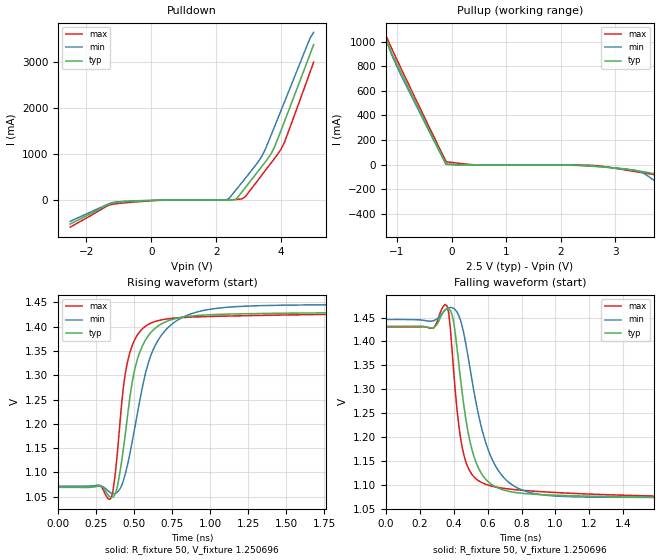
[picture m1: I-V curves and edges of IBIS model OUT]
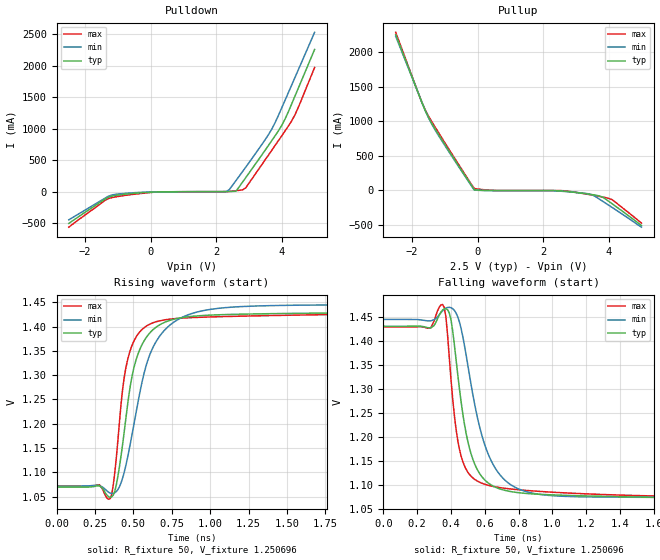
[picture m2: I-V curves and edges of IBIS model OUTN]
|   IBIS File of SG2520VGN D
|   LVDS, Vcc=2.5V, Io=3.5mA, fo<=212.5MHz
[IBIS Ver]   3.2
[File Name]   sg2520vgn_35m_25v.ibs
[File Rev]   1.0
[Date]   Sep. 11, 2020
[Source]
Fairchild Ensigna Lab's Method
[Notes]
Created by Minoru Kozaki
[Disclaimer]
Seiko Epson Corporation makes no warranty with respect to the
information contained herein.
[Copyright]
Copyright(C) 2020, Seiko Epson Corporation. All rights reserved.
|   Component
[Component]   SG2520VGN
[Manufacturer]  Seiko Epson Corporation
[Package]
R_pkg   17.7m   NA   NA
L_pkg   235p   NA   NA
C_pkg   208f   NA   NA
[Pin]   signal_name   model_name   R_pin   L_pin   C_pin
1   OE/ST   NC
2   NC   NC
3   GND   GND
4   OUT   OUT   17.7m   235p   208f
5   OUTN   OUTN   10.4m   129p   221f
6   VCC   POWER
[Diff Pin] inv_pin  vdiff  tdelay_typ
4   5   0   0
| Models and submodels in the file (2): OUT (Output), OUTN (Output)
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|   Model OUT
[Model]   OUT
Model_type   Output
Polarity   Non-Inverting
Vref = 1.25
Vmeas = 1.25
Rref = 50
Cref = 0
C_comp   4.5p   4.5p   4.5p
[Temperature Range]   25   105   -40
[Voltage Range]   2.5   2.25   2.75
[Pullup Reference]   2.5   2.25   2.75
[Pulldown Reference]   0   0   0
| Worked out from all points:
|   slope of the pulldown table from 0 to 0.375 V, typ, clamps not added: 66 ohm
|   slope of the pullup table from 0 to 0.375 V, typ, clamps not added: 55.5 ohm
|   falling waveform, R_fixture 50, V_fixture 1.250696: 20-80 % time 109ps typ, 153ps min, 81.3ps max; typ from 1.43 V to 1.07 V
|   rising waveform, R_fixture 50, V_fixture 1.250696: 20-80 % time 126ps typ, 178ps min, 93.2ps max; typ from 1.07 V to 1.43 V
[Pullup]
-2.5V     3.361A     3.265A     3.472A
-1.3V     1.161A     1.17A      1.172A
-1.2V     1.019A     1.015A     1.048A
-1V       817.6mA    797.6mA    853.4mA
-100mV    7.392mA    1.916mA    24.92mA
500mV     -3.42mA    -3.608mA   -2.547mA
2.6V      -11.61mA   -13.33mA   -5.781mA
3.4V      -49.69mA   -49.62mA   -58.4mA
3.5V      -56.25mA   -65.55mA   -65.49mA
3.8V      -93.02mA   -157.5mA   -88.11mA
4.1V      -200.5mA   -252.7mA   -132mA
5V        -521.7mA   -541.9mA   -494.1mA
[Pulldown]
-2.5V     -513.3mA   -455.2mA   -580.8mA
-1.2V     -62.9mA    -49.06mA   -86.29mA
200mV     414.9uA    905.7uA    -721.7uA
2.4V      5.862mA    46.91mA    8.441mA
2.6V      12.01mA    219mA      19.18mA
2.9V      278.6mA    480.8mA    81.84mA
3.4V      729mA      948.8mA    543mA
3.7V      1.021A     1.429A     819.6mA
4V        1.522A     1.952A     1.112A
4.1V      1.705A     2.126A     1.256A
4.8V      2.997A     3.356A     2.599A
5V        3.369A     3.636A     2.99A
[Falling Waveform]
R_fixture = 50
V_fixture = 1.250696
V_fixture_min = 1.258555
V_fixture_max = 1.251296
0s        1.432V     1.446V     1.43V
280ps     1.428V     1.443V     1.427V
360ps     1.468V     1.469V     1.474V
380ps     1.465V     1.471V     1.427V
410ps     1.414V     1.466V     1.292V
460ps     1.265V     1.415V     1.162V
540ps     1.139V     1.257V     1.11V
660ps     1.093V     1.131V     1.094V
840ps     1.081V     1.085V     1.087V
4ns       1.069V     1.071V     1.072V
[Rising Waveform]
R_fixture = 50
V_fixture = 1.250696
V_fixture_min = 1.258555
V_fixture_max = 1.251296
0s        1.069V     1.071V     1.071V
350ps     1.048V     1.057V     1.048V
400ps     1.088V     1.063V     1.176V
430ps     1.149V     1.084V     1.276V
470ps     1.249V     1.135V     1.344V
540ps     1.35V      1.252V     1.391V
650ps     1.4V       1.368V     1.412V
820ps     1.42V      1.42V      1.419V
1.15ns    1.426V     1.441V     1.422V
4ns       1.431V     1.446V     1.43V
[Ramp]
R_load = 50
dV/dt_r   0.21764/126.25p   0.22450/177.98p   0.21605/94.20p
dV/dt_f   0.21764/109.40p   0.22450/152.74p   0.21605/81.28p
|   Model OUTN
[Model]   OUTN
Model_type   Output
Polarity   Inverting
Vref = 1.25
Vmeas = 1.25
Rref = 50
Cref = 0
C_comp   4.5p   4.5p   4.5p
[Temperature Range]   25   105   -40
[Voltage Range]   2.5   2.25   2.75
[Pullup Reference]   2.5   2.25   2.75
[Pulldown Reference]   0   0   0
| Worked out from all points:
|   slope of the pulldown table from 0 to 0.375 V, typ, clamps not added: 66.2 ohm
|   slope of the pullup table from 0 to 0.375 V, typ, clamps not added: 55.6 ohm
|   falling waveform, R_fixture 50, V_fixture 1.250696: 20-80 % time 111ps typ, 154ps min, 83.9ps max; typ from 1.43 V to 1.07 V
|   rising waveform, R_fixture 50, V_fixture 1.250696: 20-80 % time 126ps typ, 179ps min, 94.5ps max; typ from 1.07 V to 1.43 V
[Pullup]
-2.5V     2.255A     2.23A      2.288A
-1.8V     1.392A     1.396A     1.397A
-1.6V     1.155A     1.16A      1.166A
-1.5V     1.054A     1.052A     1.076A
-1.3V     890.2mA    875.3mA    918.4mA
-100mV    7.351mA    1.907mA    24.74mA
500mV     -3.42mA    -3.607mA   -2.55mA
2.6V      -11.65mA   -15.29mA   -5.783mA
3.4V      -55.86mA   -52.4mA    -61.96mA
3.8V      -96.09mA   -154mA     -96.09mA
4.1V      -193.4mA   -247.2mA   -135mA
5V        -509.6mA   -533.9mA   -475.1mA
[Pulldown]
-2.5V     -499.3mA   -442.2mA   -558.6mA
-1.4V     -115.7mA   -101mA     -135.5mA
-1.2V     -68.1mA    -50.46mA   -92.45mA
200mV     410.4uA    899.3uA    -726.4uA
2.3V      4.799mA    4.53mA     5.655mA
2.4V      5.845mA    38.46mA    8.414mA
2.6V      11.95mA    179.5mA    19.06mA
2.9V      227.1mA    393.5mA    65.94mA
3.6V      743.5mA    914mA      589.8mA
4V        1.057A     1.336A     891.4mA
4.4V      1.517A     1.813A     1.222A
5V        2.259A     2.531A     1.972A
[Falling Waveform]
R_fixture = 50
V_fixture = 1.250696
V_fixture_min = 1.258555
V_fixture_max = 1.251296
0s        1.431V     1.446V     1.43V
280ps     1.428V     1.443V     1.428V
350ps     1.465V     1.464V     1.477V
370ps     1.468V     1.469V     1.451V
420ps     1.393V     1.465V     1.245V
480ps     1.226V     1.391V     1.14V
550ps     1.136V     1.251V     1.109V
670ps     1.094V     1.131V     1.095V
860ps     1.082V     1.085V     1.088V
4ns       1.07V      1.072V     1.072V
[Rising Waveform]
R_fixture = 50
V_fixture = 1.250696
V_fixture_min = 1.258555
V_fixture_max = 1.251296
0s        1.07V      1.072V     1.072V
350ps     1.048V     1.057V     1.046V
390ps     1.075V     1.061V     1.132V
430ps     1.157V     1.088V     1.27V
470ps     1.257V     1.142V     1.341V
540ps     1.352V     1.26V      1.389V
650ps     1.399V     1.37V      1.41V
820ps     1.419V     1.42V      1.418V
1.15ns    1.425V     1.44V      1.421V
4ns       1.431V     1.446V     1.43V
[Ramp]
R_load = 50
dV/dt_r   0.21660/126.56p   0.22343/177.13p   0.21502/94.97p
dV/dt_f   0.21660/110.80p   0.22343/152.89p   0.21502/83.55p
